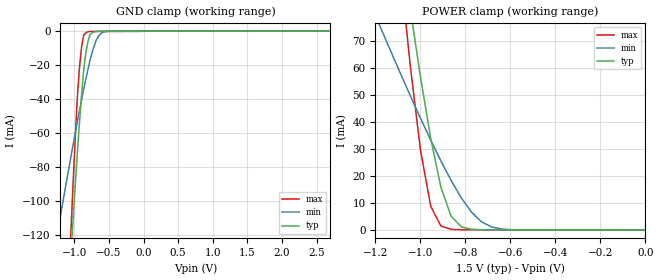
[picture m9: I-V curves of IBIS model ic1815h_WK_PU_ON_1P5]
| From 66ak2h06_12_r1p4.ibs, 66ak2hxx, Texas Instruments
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|   Model Cell ic1815h_WK_PU_ON_1P5
|WK_PU_ON_1P5
[Model]   ic1815h_WK_PU_ON_1P5
Model_type   Input
Polarity   Non-Inverting
Vinl =  0.525
Vinh =  0.975
C_comp   0.756654p   0.691399p   0.775102p
[Model Spec]
Vinl   0.525   0.4725   0.5775
Vinh   0.975   0.8775   1.0725
[Temperature Range]   25   125   -40
[Voltage Range]   1.5   1.35   1.65
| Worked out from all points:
|   GND clamp passes 1 mA (typ) near -0.74 V on its own axis
|   POWER clamp passes 1 mA (typ) near -0.81 V on its own axis
[POWER_clamp]
|   voltage   I(typ)   I(min)   I(max)
-1.5V     376.7mA    139.2mA    483.4mA
-1.182V   165.8mA    75.7mA     178.1mA
-1.167V   156.2mA    72.76mA    164.4mA
-1.061V   90.94mA    52.52mA    73.09mA
-1.03V    73.47mA    46.89mA    50.42mA
-1V       56.56mA    41.34mA    29.55mA
-954.5mV  33.86mA    33.25mA    8.795mA
-909.1mV  15.79mA    25.51mA    1.454mA
-863.6mV  5.037mA    18.29mA    246.7uA
-818.2mV  1.146mA    11.82mA    98.75uA
-681.8mV  49.7uA     1.047mA    67.68uA
0V        34.83pA    106.7pA    38.24pA
[GND_clamp]
|   voltage   I(typ)   I(min)   I(max)
-1.5V     -462.9mA   -179.8mA   -593.8mA
-1.227V   -259.3mA   -114.9mA   -299.5mA
-1.045V   -129.9mA   -73.1mA    -115.1mA
-1.015V   -109.7mA   -66.35mA   -87.58mA
-954.5mV  -70.72mA   -53.04mA   -37.87mA
-924.2mV  -53.21mA   -46.59mA   -20.98mA
-863.6mV  -22.65mA   -34.05mA   -2.371mA
-833.3mV  -13.02mA   -28.18mA   -1.11mA
-772.7mV  -2.102mA   -17.2mA    -236.1uA
-681.8mV  -196.6uA   -5.15mA    -200.2uA
-560.6mV  -118.1uA   -420.7uA   -192.1uA
3V        0A         0A         0A
